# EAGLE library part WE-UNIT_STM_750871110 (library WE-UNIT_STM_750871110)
Off-Line Transformer WE-Unit STM - Nominal input voltage: 85-265 VAC - Operating temperature: -40°C to +125 °C - Isolation voltage 4 kVAC -- Especially designed for several ICs from STMicroelectronics VIPer 28 -- Universal input -- Offline-switch mode power supplies
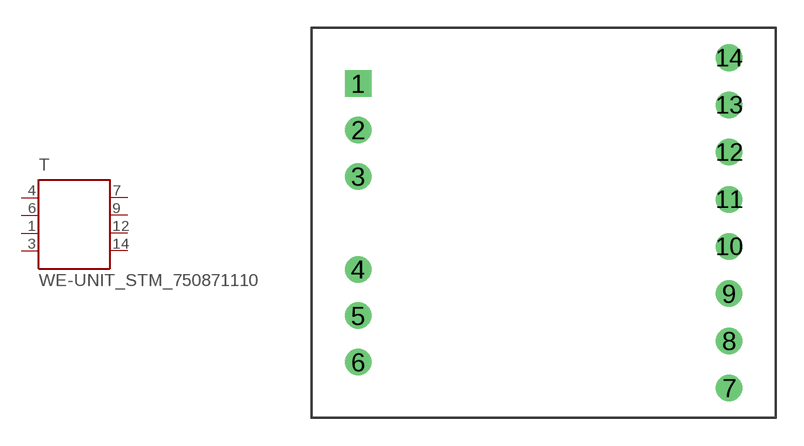
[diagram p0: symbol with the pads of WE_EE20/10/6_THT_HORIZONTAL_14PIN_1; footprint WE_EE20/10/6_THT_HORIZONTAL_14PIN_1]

Designator prefix T

## WE-UNIT_STM_750871110 (MPN: 750871110; OC_FARNELL: 1849048; OC_NEWARK: 13T9843; PACKAGE: EE20/10/6_THT_HORIZONTAL_14PIN; SUPPLIER: Würth Elektronik eiSos GmbH)  [WE_EE20/10/6_THT_HORIZONTAL_14PIN_1]
1  2  pas
3  1  pas
4  4  pas
6  3  pas
7  5  pas
9  6  pas
12  7  pas
14  8  pas

## Footprint WE_EE20/10/6_THT_HORIZONTAL_14PIN_1 (pad centres in mm)
Transformer, EE20/10/6 THT Horizontal 14Pin
drill 0.92 square: 1 -10,7.5
drill 0.92: 2 -10,5; 3 -10,2.5; 4 -10,-2.5; 5 -10,-5; 6 -10,-7.5; 7 10,-8.89; 8 10,-6.35; 9 10,-3.81; 10 10,-1.27; 11 10,1.27; 12 10,3.81; 13 10,6.35; 14 10,8.89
